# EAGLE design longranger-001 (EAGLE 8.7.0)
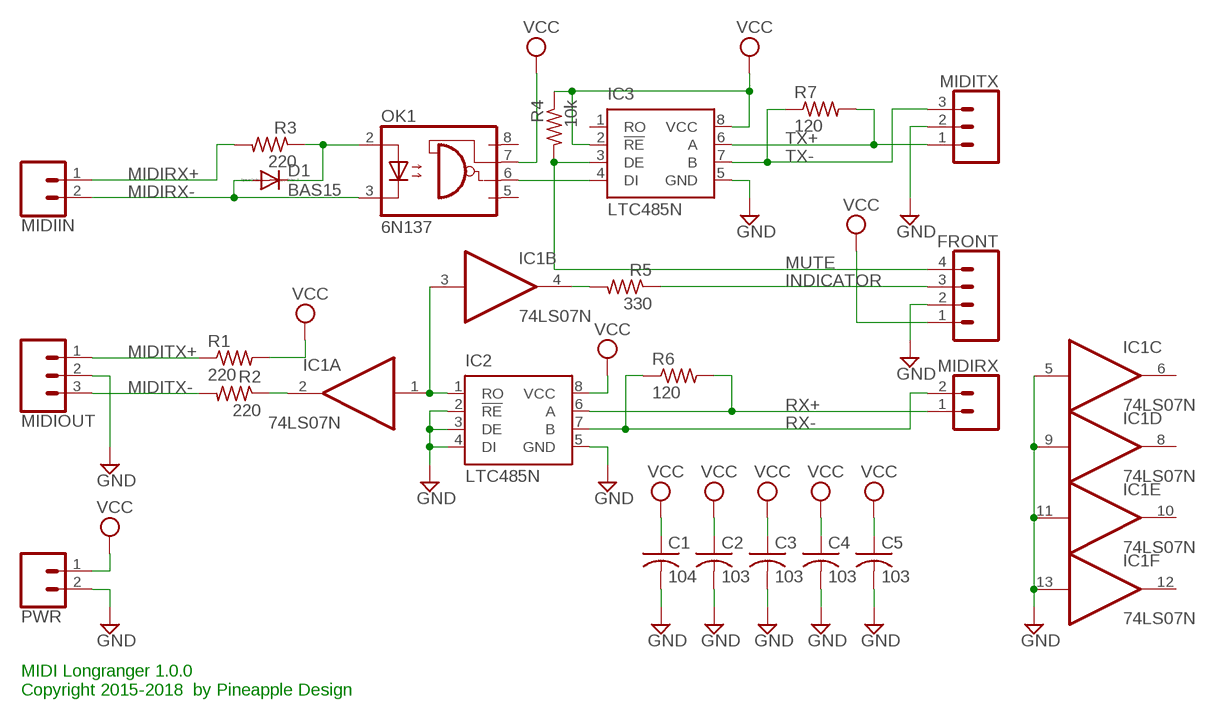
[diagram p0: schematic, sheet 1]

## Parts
C1  104  C-US025-025X050  [C025-025X050]
C2  103  C-US025-025X050  [C025-025X050]
C3  103  C-US025-025X050  [C025-025X050]
C4  103  C-US025-025X050  [C025-025X050]
C5  103  C-US025-025X050  [C025-025X050]
D1  BAS15  [DO34-7]
FRONT  CONN_04JST-PTH  [JST-4-PTH]
IC1  74LS07N  [DIL14]
IC2  LTC485N  [DIL08]
IC3  LTC485N  [DIL08]
MIDIIN  CONN_02JST-PTH-2  [JST-2-PTH]
MIDIOUT  CONN_03JST-PTH  [JST-3-PTH]
MIDIRX  CONN_02JST-PTH-2  [JST-2-PTH]
MIDITX  CONN_03JST-PTH  [JST-3-PTH]
OK1  6N137  [DIL08]
PWR  CONN_02JST-PTH-2  [JST-2-PTH]
R1  220  R-US_0204/5  [0204/5]
R2  220  R-US_0204/5  [0204/5]
R3  220  R-US_0204/5  [0204/5]
R4  10k  R-US_0204/5  [0204/5]
R5  330  R-US_0204/5  [0204/5]
R6  120  R-US_0204/5  [0204/5]
R7  120  R-US_0204/5  [0204/5]

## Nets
COM1: IC1.1(A:I) IC1.3(B:I) IC2.1(RO)
COM2: IC3.4(DI) OK1.6(VO)
GND: C1.2 C2.2 C3.2 C4.2 C5.2 FRONT.2 IC1.5(C:I) IC1.9(D:I) IC1.11(E:I) IC1.13(F:I) IC2.2(!RE) IC2.3(DE) IC2.4(DI) IC2.5(GND) IC3.5(GND) MIDIOUT.2 MIDITX.2 PWR.2
INDICATOR: FRONT.3 R5.1
MIDIRX+: MIDIIN.1 R3.2
MIDIRX-: D1.A MIDIIN.2 OK1.3(C)
MIDITX+: MIDIOUT.1 R1.1
MIDITX-: MIDIOUT.3 R2.2
MUTE: FRONT.4 IC3.3(DE) R4.2
N$2: IC1.2(A:O) R2.1
N$3: IC1.4(B:O) R5.2
N$15: D1.C OK1.2(A) R3.1
RX+: IC2.6(A) MIDIRX.1 R6.2
RX-: IC2.7(B) MIDIRX.2 R6.1
TX+: IC3.6(A) MIDITX.1 R7.2
TX-: IC3.7(B) MIDITX.3 R7.1
VCC: C1.1 C2.1 C3.1 C4.1 C5.1 FRONT.1 IC2.8(VCC) IC3.2(!RE) IC3.8(VCC) OK1.7(VE) PWR.1 R1.2 R4.1
Unconnected: IC1.6(C:O) IC1.8(D:O) IC1.10(E:O) IC1.12(F:O) IC3.1(RO) OK1.5(GND) OK1.8(VCC)

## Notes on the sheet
- MIDI Longranger 1.0.0
  Copyright 2015-2018  by Pineapple Design

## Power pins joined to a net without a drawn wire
GND: IC1.7(P:GND)
VCC: IC1.14(P:VCC)

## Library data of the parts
C1-C5 = rcl:C-US: CAPACITOR, American symbol; SPICEPREFIX: C
D1 = diode:BAS15: DIODE
FRONT = SparkFun-Connectors:CONN_04: Multi connection point. Often used as Generic Header-pin footprint for 0.1 inch spaced/style header connections On any of the 0.1 inch spaced packages, you can populate with these: Break Away Headers - Straight (PRT-00116) Break Away Male Headers - Right Angle (PRT-00553) Female Headers (PRT-00115)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; PROD_ID: WIRE-13531; SF_ID: PRT-09916
IC1 = 74xx-us:74*07: Hex BUFFER, open collector high-voltage output
IC2 IC3 = linear-technology:LTC485: Low Power RS485 Interface Transceiver Source: http://www.linear.com/pc/downloadDocument.do?navId=H0,C1,C1007,C1017,P2064,D1718; OC_FARNELL: unknown; OC_NEWARK: unknown
MIDIIN MIDIRX PWR = SparkFun-Connectors:CONN_02: Multi connection point. Often used as Generic Header-pin footprint for 0.1 inch spaced/style header connections; PROD_ID: CONN-09863; SKU: PRT-09914
MIDIOUT MIDITX = SparkFun-Connectors:CONN_03: Multi connection point. Often used as Generic Header-pin footprint for 0.1 inch spaced/style header connections On any of the 0.1 inch spaced packages, you can populate with these: Break Away Headers - Straight (PRT-00116) Break Away Male Headers - Right Angle (PRT-00553) Female Headers (PRT-00115)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; PROD_ID: WIRE-10037; SF_ID: PRT-09915
OK1 = optocoupler:6N137: MOTOROLA OPTO COUPLER; MPN: 6N137; OC_FARNELL: 1328376; OC_NEWARK: 52M1895
R1-R7 = resistor:R-US_: RESISTOR, American symbol

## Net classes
0 default: width 0.254 mm, drill 0.254 mm, clearance 0.254 mm

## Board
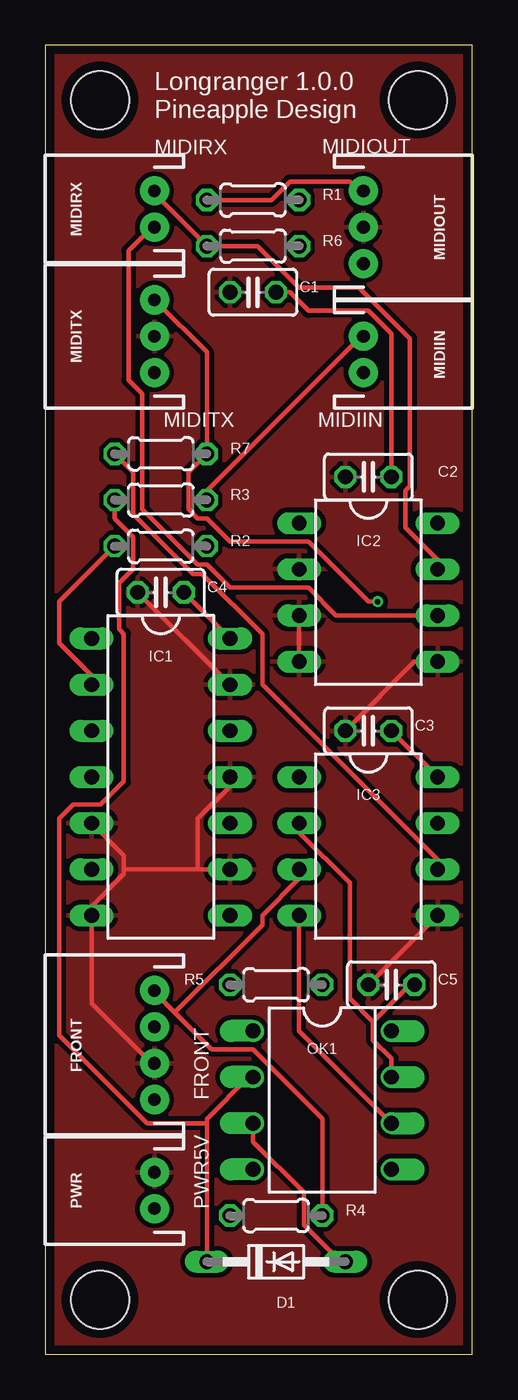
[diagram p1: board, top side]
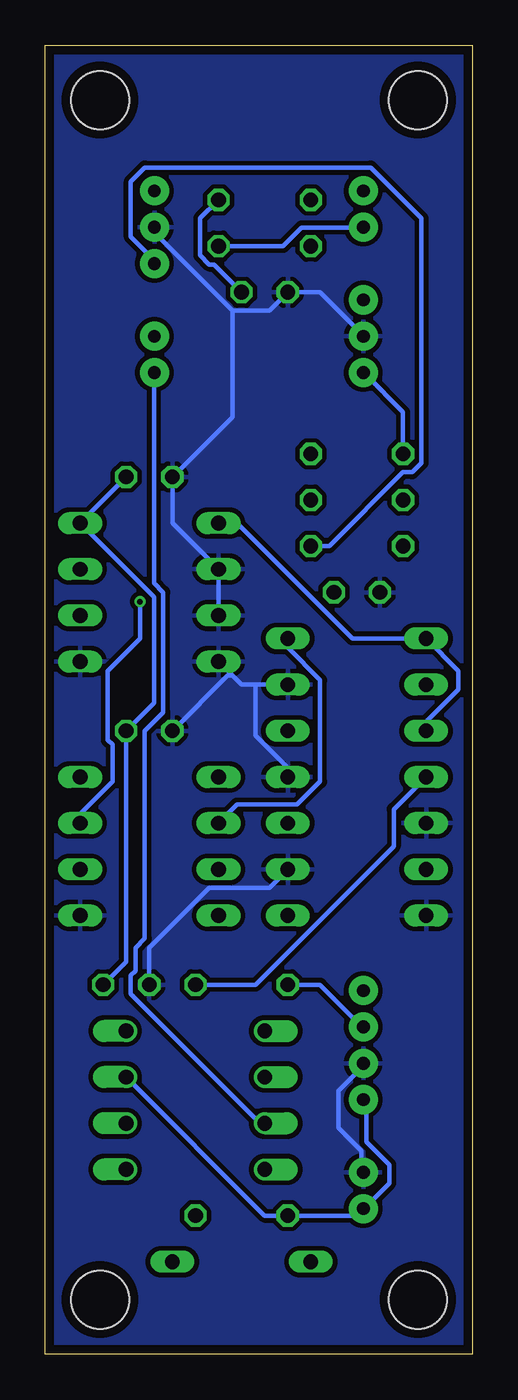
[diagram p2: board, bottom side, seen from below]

Size 23.5 x 72 mm. Coordinates in mm from the lower left corner, seen from the top.
Outline: 0,0 23.5,0 23.5,72 0,72 0,0
Copper layers (1*16): Top 0.035mm / dielectric 1.53mm / Bottom 0.035mm
Design rules "pban_5mil-l2 *": minimum track width 5mil, minimum drill 0.3mm, track to track 10mil, track to pad 10mil, pad to pad 10mil, via to via 10mil, smd to smd 5mil, copper to edge 0.5mm, drill to drill 0.5mm, minimum pad ring 0.15mm, minimum via ring 0.15mm, stop-mask expansion 4mil, vias tented up to drill 0.35mm, thermal gap 10mil
Holes 3.2 mm at 3,3 20.5,3 20.5,69 3,69

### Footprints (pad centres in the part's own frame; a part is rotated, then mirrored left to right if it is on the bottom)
C025-025X050 = drill 0.813 octagon: 1 -1.27,0; 2 1.27,0
DO34-7 = drill 0.813 long: A 3.81,0; C -3.81,0
JST-4-PTH = drill 0.7 pad 1.6: 1 -3,0; 2 -1,0; 3 1,0; 4 3,0
DIL14 = drill 0.813 long: 1 -7.62,-3.81; 2 -5.08,-3.81; 3 -2.54,-3.81; 4 0,-3.81; 5 2.54,-3.81; 6 5.08,-3.81; 7 7.62,-3.81; 8 7.62,3.81; 9 5.08,3.81; 10 2.54,3.81; 11 0,3.81; 12 -2.54,3.81; 13 -5.08,3.81; 14 -7.62,3.81
DIL08 = drill 0.813 long: 1 -3.81,-3.81; 2 -1.27,-3.81; 3 1.27,-3.81; 4 3.81,-3.81; 5 3.81,3.81; 6 1.27,3.81; 7 -1.27,3.81; 8 -3.81,3.81
JST-2-PTH = drill 0.7 pad 1.6: 1 -1,0; 2 1,0
JST-3-PTH = drill 0.7 pad 1.6: 1 -2,0; 2 0,0; 3 2,0
DIL08' = drill 0.813 offset: 1 -3.81,-3.81; 2 -1.27,-3.81; 3 1.27,-3.81; 4 3.81,-3.81; 5 3.81,3.81; 6 1.27,3.81; 7 -1.27,3.81; 8 -3.81,3.81
0204/5 = drill 0.813 octagon: 1 -2.54,0; 2 2.54,0

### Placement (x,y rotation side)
C1  11.43,58.42 180 top
C2  17.78,48.26 180 top
C3  17.78,34.29 180 top
C4  6.35,41.91 180 top
C5  19.05,20.32 180 top
D1  12.7,5.08 0 top
FRONT  6,17 90 top
IC1  6.35,31.75 270 top
IC2  17.78,41.91 270 top
IC3  17.78,27.94 270 top
MIDIIN  17.5,55 270 top
MIDIOUT  17.5,62 270 top
MIDIRX  6,63 90 top
MIDITX  6,56 90 top
OK1  6N137  [DIL08']  15.24,13.97 270 top
PWR  6,9 90 top
R1  11.43,63.5 0 top
R2  6.35,44.45 0 top
R3  6.35,46.99 0 top
R4  12.7,7.62 0 top
R5  12.7,20.32 0 top
R6  11.43,60.96 0 top
R7  6.35,49.53 180 top

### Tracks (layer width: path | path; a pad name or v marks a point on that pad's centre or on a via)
COM1
  Bottom 0.254: IC1.3 2.54,34.8 0.76,36.58 0.76,37.59 IC1.1 6.6,39.37 12.95,45.72 IC2.1
COM2
  Top 0.254: IC3.4 13.97,17.78 OK1.6
GND
  Top 0.254: IC3.5 C5.2 | 4.32,26.67 4.32,27.43 IC1.5 | 4.32,26.67 4.32,26.42 2.54,24.64 IC1.7 2.54,19.3 5.84,16 FRONT.2 | 4.32,26.67 8.38,26.67 | 8.38,26.67 IC1.9 | IC1.11 10.16,31.24 8.38,29.46 8.38,26.67 | IC1.13 C4.2 | IC2.4 IC2.3 | IC2.5 20.32,38.1 C3.2
  Bottom 0.254: PWR.2 6.1,10.16 6.1,11.18 7.37,12.45 7.37,14.48 6.1,15.75 FRONT.2 | C5.2 17.78,22.35 14.48,25.65 11.18,25.65 IC1.9 | MIDITX.2 6.1,56.13 8.38,58.42 C1.2 11.18,57.4 13.21,57.4 | 13.21,57.4 17.27,61.47 17.27,61.98 MIDIOUT.2 | 11.94,36.83 12.7,36.83 13.21,37.34 | 11.94,36.83 IC1.13 | IC2.4 13.21,37.34 | C3.2 13.46,37.34 13.21,37.34 | IC2.3 IC2.2 16.51,45.72 C2.2 13.21,51.56 13.21,57.4 | IC1.11 10.16,32.26 11.94,34.04 11.94,36.83
  pour Top (isolate 0.254): 0,0 23.5,0 23.5,72 0.5,72 0,72
  pour Bottom (isolate 0.254): 0,0 23.5,0 23.5,72 0,72
INDICATOR
  Bottom 0.254: R5.1 8.38,20.32 6.1,18.03 FRONT.3
MIDIRX+
  Top 0.254: R3.2 8.89,47.5 17.27,55.88 MIDIIN.1
MIDIRX-
  Top 0.254: OK1.3 11.43,11.68 14.22,8.89 14.22,7.11 16.26,5.08 D1.A
  Bottom 0.254: OK1.3 11.68,12.7 18.8,19.81 18.8,20.83 18.54,21.08 18.54,22.35 18.03,22.86 18.03,34.29 17.02,35.31 17.02,41.91 17.53,42.42 17.53,53.85 MIDIIN.2
MIDITX+
  Top 0.254: R1.1 12.45,63.5 13.46,64.52 16.76,64.52 17.27,64.01 MIDIOUT.1
MIDITX-
  Bottom 0.254: R2.2 7.87,44.45 3.81,48.51 3.3,48.51 2.79,49.02 2.79,62.48 5.59,65.28 18.03,65.28 18.8,64.52 18.8,61.47 17.53,60.2 MIDIOUT.3
MUTE
  Top 0.254: R4.2 15.24,12.95 11.43,16.76 9.14,16.76 7.11,18.8 | 7.11,18.8 6.1,19.81 FRONT.4 | IC3.3 13.97,26.16 11.94,24.13 11.94,23.62 7.11,18.8
N$2
  Top 0.254: IC1.2 2.54,37.34 0.76,39.12 0.76,41.4 R2.1
N$3
  Bottom 0.254: R5.2 11.94,20.32 4.32,27.94 4.32,29.97 IC1.4
N$15
  Top 0.254: 8.89,12.7 8.89,12.95 11.18,15.24 OK1.2 | 8.89,12.7 D1.C | R3.1 3.81,45.97 4.83,44.96 4.83,43.18 4.06,42.42 4.06,39.88 4.32,39.62 4.32,31.5 3.05,30.23 1.52,30.23 0.76,29.46 0.76,17.53 5.59,12.7 8.89,12.7
RX+
  Top 0.254: IC2.6 16,40.64 14.48,42.16 10.16,42.16 8.89,43.43 8.38,43.43 5.33,46.48 5.33,52.83 4.57,53.59 4.57,60.71 5.84,61.98 MIDIRX.1
  Bottom 0.254: R6.2 10.41,60.96 9.4,61.98 6.1,61.98 MIDIRX.1
RX-
  Top 0.254: MIDIRX.2 6.1,63.75 R6.1 11.68,60.96 13.97,58.67 17.27,58.67 20.07,55.88 20.07,47.75 19.81,47.5 19.81,45.47 21.59,43.69 IC2.7
TX+
  Top 0.254: IC3.6 21.59,27.18 11.94,36.83 11.94,39.62 8.64,42.93 8.13,42.93 4.83,46.23 4.83,48.51 R7.2
  Bottom 0.254: R7.2 3.81,51.82 5.84,53.85 MIDITX.1
TX-  (via drill 0.3)
  Top 0.254: MIDITX.3 6.1,57.91 8.89,55.12 R7.1 7.87,48.51 7.87,46.48 8.38,45.97 8.89,45.97 10.16,44.7 14.48,44.7 17.78,41.4 v18.29,41.4
  Bottom 0.254: IC3.7 21.59,29.72 19.81,31.5 19.81,33.53 20.07,33.78 20.07,37.59 18.29,39.37 v18.29,41.4
VCC
  Top 0.254: C4.1 IC1.14 | IC3.8 C3.1 | OK1.7 19.05,16.26 18.03,17.27 18.03,18.29 | 18.03,18.29 20.07,20.32 C5.1 | IC3.2 13.97,28.7 16.76,25.91 16.76,19.56 18.03,18.29 | C1.1 13.46,58.42 14.48,57.4 17.78,57.4 19.05,56.13 C2.1
  Bottom 0.254: FRONT.1 5.84,13.97 5.84,11.68 4.57,10.41 4.57,9.4 5.84,8.13 PWR.1 6.1,7.87 6.35,7.62 R4.1 11.43,7.62 OK1.7 | C1.1 14.22,59.94 14.48,59.94 14.99,60.45 14.99,62.48 R1.2 | C2.1 IC2.8 17.53,41.66 17.53,35.81 C3.1 19.05,21.59 C5.1 | IC1.14 10.16,38.86 8.38,37.08 8.38,31.5 9.65,30.23 12.95,30.23 IC3.2

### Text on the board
tNames: Longranger 1.0.0 / Pineapple Design | MIDIRX | MIDIOUT | MIDITX | MIDIIN | FRONT | PWR5V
